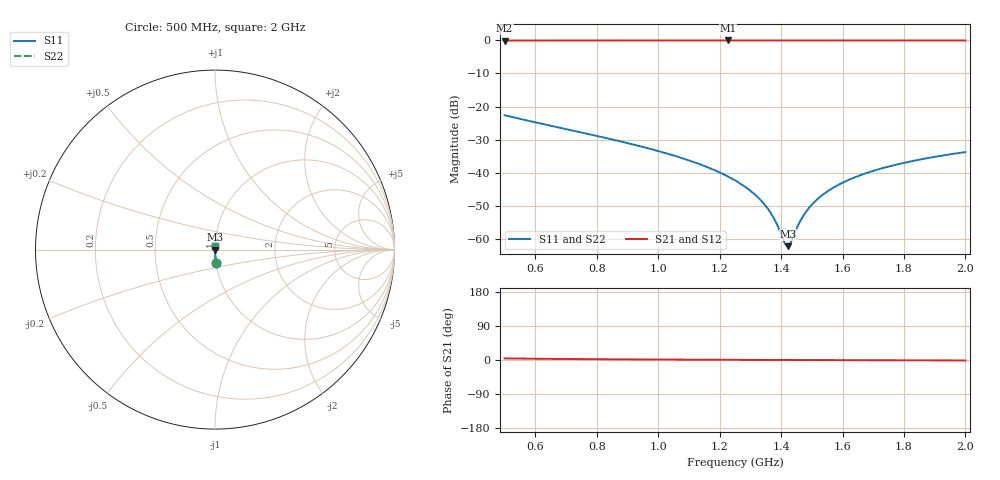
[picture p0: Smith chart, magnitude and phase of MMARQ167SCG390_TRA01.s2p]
! MMARQ167SCG390_TRA01  S-PARAMETER MODEL  ( General Type )
! Model Generated by TAIYO YUDEN Corporation (http://www.ty-top.com)
! Version 1.0
! TAIYO YUDEN Control No. 150305
! Copyright(c) 2015 TAIYO YUDEN CO.,LTD. All Rights Reserved.
! Product Description (link to TY-COMPAS)
! https://ds.yuden.co.jp/TYCOMPAS/or/detail?pn=MMARQ167SCG390JTRA01&u=M
! Products Name : Multilayer Ceramic Capacitors
! Characteristics :
!  Capacitance : 39 pF , Rated Voltage : 250V , TCC : CG / C0G
!  Case Size : 1.6 x 0.8 / 0.063 x 0.031 [mm/inch] , Thickness : 0.7 / 0.028 [mm/inch]
!  (Conditions: Temperature = 25 degC , DC Bias Current/Voltage = 0A / 0V)
! External Node Assignments :
!  1  o---| |---o  2
! GND o---------o GND
! Frequency Range : 500MHz  -  2GHz  [ 401 STEP ]
# MHz S RI R 50
! Freq[MHz].  S11 Real  S11 Imag  S21 Real  S21 Imag  S12 Real  S12 Imag  S22 Real  S22 Imag
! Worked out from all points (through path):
!   401 points, 500 MHz to 2 GHz, reference 50 ohm
!   highest |S21| = -0.01 dB at 1.228 GHz (marker M1); lowest = 0.0 dB at 500 MHz (marker M2)
!   lowest |S11| = -62.2 dB at 1.423 GHz (marker M3), VSWR 1.00, Z = 50.1 + j0.00433 ohm
!   |S11| at or under -10 dB: start of sweep to end of sweep
!   |S22| runs from -62.2 to -22.6 dB; largest |S21 - S12| = 0
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500  0.00576 -0.0736  0.9942 0.0736  0.9942 0.0736  0.00576 -0.0736
751.25  0.00209 -0.0403  0.9979 0.0403  0.9979 0.0403  0.00209 -0.0403
1002.5  0.00104 -0.0211  0.999 0.0211  0.999 0.0211  0.00104 -0.0211
1130  0.000838 -0.0137  0.9992 0.0137  0.9992 0.0137  0.000838 -0.0137
1227.5  0.000769 -0.00869  0.9992 0.00869  0.9992 0.00869  0.000769 -0.00869
1250  0.000761 -0.00761  0.9992 0.00761  0.9992 0.00761  0.000761 -0.00761
1306.25  0.000751 -0.00499  0.9992 0.00499  0.9992 0.00499  0.000751 -0.00499
1347.5  0.000752 -0.00315  0.9992 0.00315  0.9992 0.00315  0.000752 -0.00315
1377.5  0.000757 -0.00185  0.9992 0.00185  0.9992 0.00185  0.000757 -0.00185
1411.25  0.000767 -0.000425  0.9992 0.000425  0.9992 0.000425  0.000767 -0.000425
1418.75  0.000769 -0.000112  0.9992 0.000112  0.9992 0.000112  0.000769 -0.000112
1422.5  0.000771 4.32e-05  0.9992 -4.32e-05  0.9992 -4.32e-05  0.000771 4.32e-05
1433.75  0.000775 0.000507  0.9992 -0.000507  0.9992 -0.000507  0.000775 0.000507
1452.5  0.000783 0.00127  0.9992 -0.00127  0.9992 -0.00127  0.000783 0.00127
1467.5  0.000791 0.00188  0.9992 -0.00188  0.9992 -0.00188  0.000791 0.00188
1501.25  0.00081 0.00322  0.9992 -0.00322  0.9992 -0.00322  0.00081 0.00322
1542.5  0.000837 0.00482  0.9992 -0.00482  0.9992 -0.00482  0.000837 0.00482
1598.75  0.000881 0.00694  0.9991 -0.00694  0.9991 -0.00694  0.000881 0.00694
1666.25  0.000942 0.00939  0.9991 -0.00939  0.9991 -0.00939  0.000942 0.00939
1752.5  0.00103 0.0124  0.999 -0.0124  0.999 -0.0124  0.00103 0.0124
1868.75  0.00118 0.0163  0.9988 -0.0163  0.9988 -0.0163  0.00118 0.0163
2000  0.00137 0.0204  0.9986 -0.0204  0.9986 -0.0204  0.00137 0.0204
